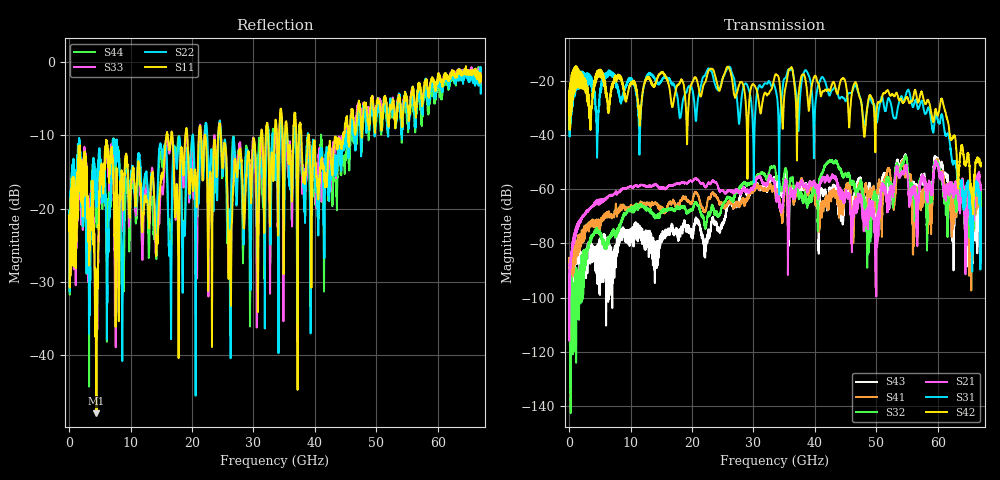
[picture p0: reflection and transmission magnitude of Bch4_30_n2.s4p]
!Agilent Technologies,N5247A,US51170199,A.09.90.13
!Agilent N5247A: A.09.90.13
!Date: Wednesday, October 17, 2018 18:02:45
!Correction: S11(Full 4 Port(1,2,3,4))
!S12(Full 4 Port(1,2,3,4))
!S13(Full 4 Port(1,2,3,4))
!S14(Full 4 Port(1,2,3,4))
!S21(Full 4 Port(1,2,3,4))
!S22(Full 4 Port(1,2,3,4))
!S23(Full 4 Port(1,2,3,4))
!S24(Full 4 Port(1,2,3,4))
!S31(Full 4 Port(1,2,3,4))
!S32(Full 4 Port(1,2,3,4))
!S33(Full 4 Port(1,2,3,4))
!S34(Full 4 Port(1,2,3,4))
!S41(Full 4 Port(1,2,3,4))
!S42(Full 4 Port(1,2,3,4))
!S43(Full 4 Port(1,2,3,4))
!S44(Full 4 Port(1,2,3,4))
!S4P File: Measurements: <S11,S12,S13,S14>,
!<S21,S22,S23,S24>,
!<S31,S32,S33,S34>,
!<S41,S42,S43,S44>:
# Hz S  dB  R 50
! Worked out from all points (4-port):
!   6701 points, 10 MHz to 67 GHz, reference 50 ohm
!   strongest paths, dB at 10 MHz, 16.76 GHz, 33.51 GHz, 50.25 GHz, 67 GHz:
!     S42: -32.3, -29.5, -17.9, -28.0, -51.5
!     S31: -32.6, -21.2, -22.4, -33.0, -69.0
!     S21: -87.7, -58.7, -58.6, -70.1, -58.5
!     S32: -90.0, -67.1, -52.0, -72.3, -67.9
!     S41: -85.3, -65.0, -60.2, -59.6, -64.5
!     S43: -92.6, -74.2, -56.6, -65.2, -73.6
!   lowest |S11| = -47.9 dB at 4.459 GHz (marker M1), VSWR 1.01, Z = 50.1 - j0.396 ohm
!   |S11| at or under -10 dB: start of sweep to 15.82 GHz; 24.69 GHz to 31.22 GHz (6.53 GHz wide, 23.4 % of centre); 39.03 GHz to 44.62 GHz (5.586 GHz wide, 13.4 % of centre)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
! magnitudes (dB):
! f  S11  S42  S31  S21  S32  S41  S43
! 10 MHz  -23.0  -32.3  -32.6  -87.7  -90.0  -85.3  -92.6
! 4.459 GHz  -47.9  -18.9  -34.6  -64.0  -74.4  -71.6  -90.9
! 6.049 GHz  -10.8  -25.7  -17.3  -63.6  -80.2  -68.8  -83.6
! 42.62 GHz  -13.9  -22.2  -23.9  -55.7  -49.5  -62.5  -62.3
! 48.74 GHz  -8.7  -26.3  -27.2  -68.4  -69.7  -68.0  -58.8
! 55.14 GHz  -6.5  -26.7  -23.3  -57.6  -52.8  -54.7  -54.9
! 67 GHz  -2.6  -51.5  -69.0  -58.5  -67.9  -64.5  -73.6
